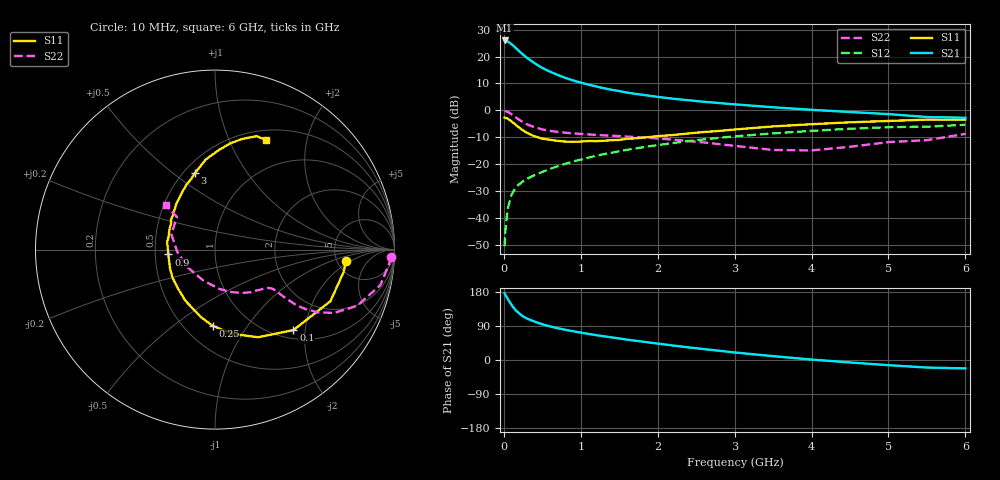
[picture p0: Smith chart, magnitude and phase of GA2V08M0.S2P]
! Infineon Technologies  Discrete & RF Semiconductors
! BF775
! Si NPN RF Bipolar Junction Transistor in SOT23
! VCE = 2 V  IC = 8 mA
! Common Emitter S-Parameters:  May  1996
# GHz  S  MA  R  50
!  f  S11  S21  S12  S22
! GHz  MAG  ANG  MAG  ANG  MAG  ANG  MAG  ANG
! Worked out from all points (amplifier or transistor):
!   36 points, 10 MHz to 6 GHz, reference 50 ohm
!   highest |S21| = 26.0 dB at 10 MHz (marker M1)
!   |S21| within 3 dB of that: start of sweep to 162.5 MHz
!   unconditionally stable (mu >= 1): 610 MHz to 3.823 GHz
!   at 250 MHz: K = 0.63, MSG = 23.5 dB, |S12| = -26.3 dB
!   at 1.4 GHz: K = 1.14, MAG = 9.5 dB, |S12| = -15.7 dB
!   at 6 GHz: K = 0.98, MSG = 1.3 dB, |S12| = -5.3 dB
!   S11 on the Smith chart (normalised r, x): 10 MHz: 6.03, -1.67; 100 MHz: 1.17, -1.73; 250 MHz: 0.68, -0.70; 900 MHz: 0.59, -0.03; 3 GHz: 0.57, +0.60; 6 GHz: 0.62, +1.38
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0.01  0.7335 -5.0  19.95 176.2  0.003 89.5  0.9833 -2.4
0.02  0.7268 -10.1  19.85 172.0  0.0058 84.8  0.972 -5.0
0.05  0.7045 -24.1  19.12 161.3  0.0149 77.6  0.9423 -12.1
0.1  0.6259 -45.8  17.09 145.3  0.0271 69.2  0.8514 -21.6
0.15  0.5441 -63.8  14.65 132.1  0.036 63.6  0.7515 -28.0
0.2  0.4795 -78.3  12.62 122.8  0.0425 60.4  0.6707 -31.4
0.25  0.4247 -91.8  10.88 115.2  0.0484 58.7  0.6036 -33.3
0.3  0.3838 -101.8  9.498 109.5  0.0535 58.6  0.5525 -34.3
0.4  0.3299 -119.7  7.527 101.2  0.0629 58.8  0.4868 -34.5
0.5  0.2984 -134.2  6.158 94.2  0.0719 59.6  0.4437 -34.4
0.6  0.2845 -146.1  5.245 88.7  0.0821 60.2  0.4167 -34.1
0.7  0.2717 -157.3  4.563 83.9  0.0918 60.8  0.3984 -34.1
0.9  0.2611 -174.0  3.602 75.9  0.1124 61.0  0.3742 -35.0
1.1  0.27 171.1  3.017 68.9  0.1326 60.6  0.3583 -37.1
1.3  0.2729 159.6  2.586 62.6  0.1539 59.7  0.3444 -39.3
1.6  0.2972 145.5  2.149 53.7  0.1849 57.6  0.3257 -44.3
2.2  0.3492 124.7  1.649 38.2  0.2476 51.7  0.2872 -57.2
3  0.4414 104.6  1.296 19.9  0.3289 42.1  0.2196 -84.1
3.5  0.5042 95.9  1.143 10.1  0.3742 35.5  0.1839 -111.2
4.5  0.6006 81.5  0.934 -6.5  0.4563 22.0  0.2105 -176.4
5.5  0.6741 69.7  0.753 -19.9  0.4988 7.6  0.2799 139.3
6  0.6719 64.8  0.73 -22.2  0.5405 3.6  0.3668 137.9
